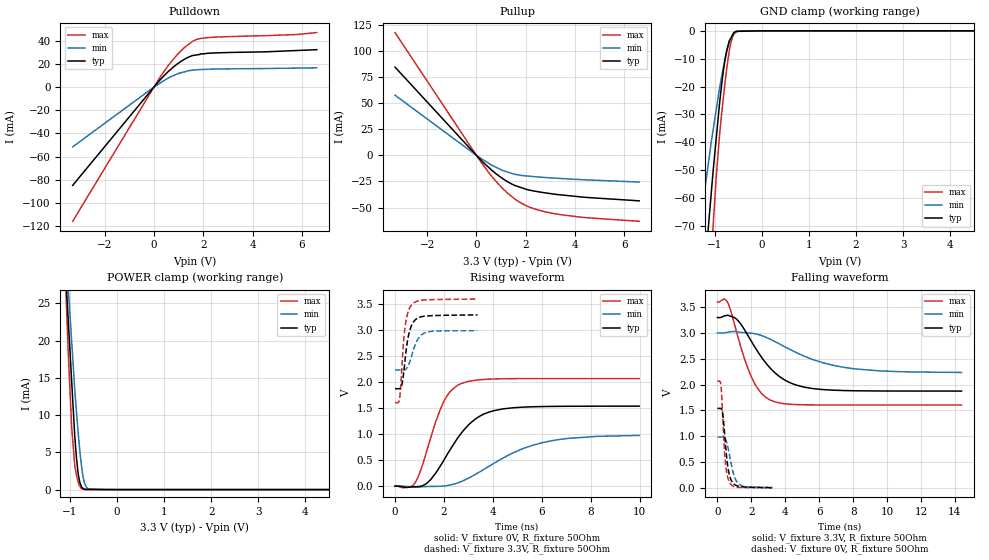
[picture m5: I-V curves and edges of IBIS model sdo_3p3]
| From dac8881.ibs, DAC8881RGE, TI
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|   sdo_3p3 Model
[Model]   sdo_3p3
Model_type   3-state
Polarity   Non-Inverting
Vmeas = 1.65
Vref = 1.65
Cref = 50pF
Rref = 50
|   typ   min   max
|   (nom PVT)   (fast PVT)   (slow PVT)
|C_comp from frequency sweep method (F=25MHz)
|C_comp   6.287e-12   5.236e-12   7.628e-12
|ON state : BUFFER OUTPUT TURNED HIGH
|C_comp   6.287e-12   5.236e-12   7.628e-12
|OFF state: BUFFER IN HIGH IMPEDANCE
|C_comp   3.684e-12   2.864e-12   4.477e-12
|C_comp from LC tank measurement(L=1nH)
|Resonant Frequency(Hz)   2.880e+09   3.150e+09   2.660e+09
|C_comp   3.057e-12   2.555e-12   3.584e-12
|ON state : BUFFER OUTPUT TURNED HIGH
|Resonant Frequency(Hz)   2.880e+09   3.150e+09   2.660e+09
|C_comp   3.057e-12   2.555e-12   3.584e-12
|OFF state: BUFFER IN HIGH IMPEDANCE
|Resonant Frequency(Hz)   2.950e+09   3.260e+09   2.710e+09
C_comp   2.914e-12   2.386e-12   3.452e-12
| Where nom  PVT is Nominal Process, 3.3V, 25C
|   Fast PVT is Strong Process,  3.6V, -40C
|   Slow PVT is Weak Process,   3V, 105C
[Voltage Range]   3.3   3   3.6
|Ambient Temperature   25   105   -40
|Junction Temperature
[Temperature Range]   25   105   -40
[Pullup Reference]   3.3   3   3.6
[Pulldown Reference]   0   0   0
[Power Clamp Reference]   3.3   3   3.6
[GND Clamp Reference]   0   0   0
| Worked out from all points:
|   slope of the pulldown table from 0 to 0.495 V, typ, clamps not added: 42.9 ohm
|   slope of the pullup table from 0 to 0.495 V, typ, clamps not added: 43.1 ohm
|   GND clamp passes 1 mA (typ) near -0.60 V on its own axis
|   POWER clamp passes 1 mA (typ) near -0.79 V on its own axis
|   falling waveform, V_fixture 3.3V, R_fixture 50Ohm: 20-80 % time 1.96ns typ, 3.33ns min, 1.25ns max; typ from 3.3 V to 1.88 V
|   rising waveform, V_fixture 0V, R_fixture 50Ohm: 20-80 % time 1.39ns typ, 2.42ns min, 898ps max; typ from 0 V to 1.54 V
|   rising waveform, V_fixture 3.3V, R_fixture 50Ohm: 20-80 % time 265ps typ, 355ps min, 212ps max; typ from 1.88 V to 3.3 V
|   falling waveform, V_fixture 0V, R_fixture 50Ohm: 20-80 % time 288ps typ, 398ps min, 222ps max; typ from 1.54 V to 0.005 V
[Pulldown]
|   Voltage   I(typ)   I(min)   I(max)
-3.3V     -84.83mA   -51.69mA   -115.8mA
172.8mV   4.34mA     2.365mA    5.975mA
651.6mV   14.72mA    8.575mA    20.52mA
939.6mV   19.77mA    11.18mA    27.79mA
1.246V    24.05mA    13.11mA    34.24mA
1.573V    27.13mA    14.54mA    39.48mA
1.814V    27.9mA     14.94mA    41.49mA
2.012V    28.53mA    15.13mA    42.2mA
5.774V    31.41mA    16.27mA    45.18mA
6.6V      32.15mA    16.53mA    46.89mA
[GND Clamp]
|   Voltage   I(typ)   I(min)   I(max)
-3.3V     -574.6mA   -389.1mA   -790mA
-1.368V   -119.7mA   -77.83mA   -170.9mA
-1.272V   -99.15mA   -64.97mA   -141.8mA
-1.201V   -84.02mA   -56.1mA    -120.4mA
-1.071V   -58.06mA   -39.83mA   -80.98mA
-1.033V   -50.46mA   -35.65mA   -70.2mA
-896.4mV  -26.21mA   -20.68mA   -37.57mA
-784.8mV  -10.91mA   -10.65mA   -19.41mA
-693mV    -3.752mA   -4.477mA   -7.669mA
-655.2mV  -2.584mA   -2.973mA   -4.325mA
-544.5mV  -199.5uA   -445.9uA   -403.7uA
6.6V      0A         0A         0A
[Pullup]
|   Voltage   I(typ)   I(min)   I(max)
-3.3V     84.43mA    57.59mA    117.5mA
172.8mV   -4.272mA   -2.682mA   -6.008mA
583.2mV   -13.38mA   -8.913mA   -18.99mA
939.6mV   -20.19mA   -13.06mA   -28.71mA
1.246V    -24.99mA   -15.83mA   -35.81mA
1.588V    -29.1mA    -18.24mA   -42.32mA
2.167V    -33.36mA   -19.98mA   -49.72mA
3.089V    -36.92mA   -21.67mA   -55.5mA
4.496V    -40.34mA   -23.51mA   -59.74mA
6.6V      -43.54mA   -25.57mA   -63.12mA
[POWER Clamp]
|   Voltage   I(typ)   I(min)   I(max)
-3.3V     228.6mA    199.5mA    263.7mA
-1.454V   76.97mA    68.62mA    90.17mA
-1.059V   25.49mA    29.54mA    22.54mA
-1.037V   22.97mA    27.32mA    18.74mA
-961.2mV  14.48mA    19.84mA    8.312mA
-896.4mV  7.233mA    13.44mA    3.232mA
-858mV    4.132mA    10.25mA    1.856mA
-821.7mV  2.062mA    7.462mA    1.011mA
-738mV    254.3uA    2.458mA    66.72uA
-681mV    39.15uA    730.5uA    7.098uA
-591mV    33.95uA    58.88uA    1.4uA
6.6V      0A         0A         0A
[Ramp]
R_load = 50
|   typ   min   max
dV/dt_r   0.924394/1.37952e-09   0.591221/2.45502e-09   1.24237/8.97677e-10
dV/dt_f   0.854356/1.95788e-09   0.459397/3.33779e-09   1.19615/1.24471e-09
[Falling Waveform]
V_fixture = 3.3V
V_fixture_min = 3V
V_fixture_max = 3.6V
R_fixture = 50Ohm
|   Time   V(typ)   V(min)   V(max)
0s        3.3V       3V         3.6V
415ps     3.332V     3.002V     3.657V
625ps     3.344V     3.017V     3.579V
1.265ns   3.223V     3.017V     2.862V
1.95ns    2.87V      2.998V     2.191V
2.565ns   2.548V     2.956V     1.845V
3.205ns   2.289V     2.866V     1.69V
4.65ns    1.992V     2.621V     1.614V
7.425ns   1.886V     2.337V     1.606V
14.39ns   1.876V     2.237V     1.606V
[Rising Waveform]
V_fixture = 0V
V_fixture_min = 0V
V_fixture_max = 0V
R_fixture = 50Ohm
|   Time   V(typ)   V(min)   V(max)
0s        1.148nV    1.426nV    1.035nV
820ps     -9.142mV   -17.83mV   66.91mV
1.295ns   56.33mV    -5.914mV   674.8mV
1.945ns   460.6mV    2.202mV    1.581V
2.245ns   697.6mV    22.17mV    1.815V
2.695ns   1.014V     88.28mV    1.975V
3.445ns   1.343V     271.3mV    2.047V
4.385ns   1.485V     534.8mV    2.068V
6.53ns    1.536V     886mV      2.071V
9.975ns   1.54V      977.5mV    2.071V
[Rising Waveform]
V_fixture = 3.3V
V_fixture_min = 3V
V_fixture_max = 3.6V
R_fixture = 50Ohm
|   Time   V(typ)   V(min)   V(max)
0s        1.876V     2.234V     1.606V
175ps     1.876V     2.234V     1.662V
235ps     1.896V     2.234V     1.94V
290ps     1.979V     2.234V     2.371V
410ps     2.428V     2.241V     3.059V
525ps     2.837V     2.306V     3.341V
670ps     3.088V     2.496V     3.485V
925ps     3.234V     2.822V     3.562V
1.24ns    3.273V     2.956V     3.584V
3.37ns    3.296V     2.993V     3.599V
[Falling Waveform]
V_fixture = 0V
V_fixture_min = 0V
V_fixture_max = 0V
R_fixture = 50Ohm
|   Time   V(typ)   V(min)   V(max)
0s        1.54V      985.3mV    2.068V
155ps     1.54V      985.1mV    2.062V
215ps     1.538V     985.2mV    1.962V
310ps     1.436V     987.1mV    1.409V
440ps     990.2mV    968.3mV    608.8mV
540ps     613.9mV    893.7mV    311.3mV
680ps     289.3mV    692.1mV    132.5mV
965ps     77.11mV    254.7mV    27.29mV
1.255ns   32.04mV    77.21mV    10.32mV
3.25ns    4.821mV    9.726mV    1.118mV
